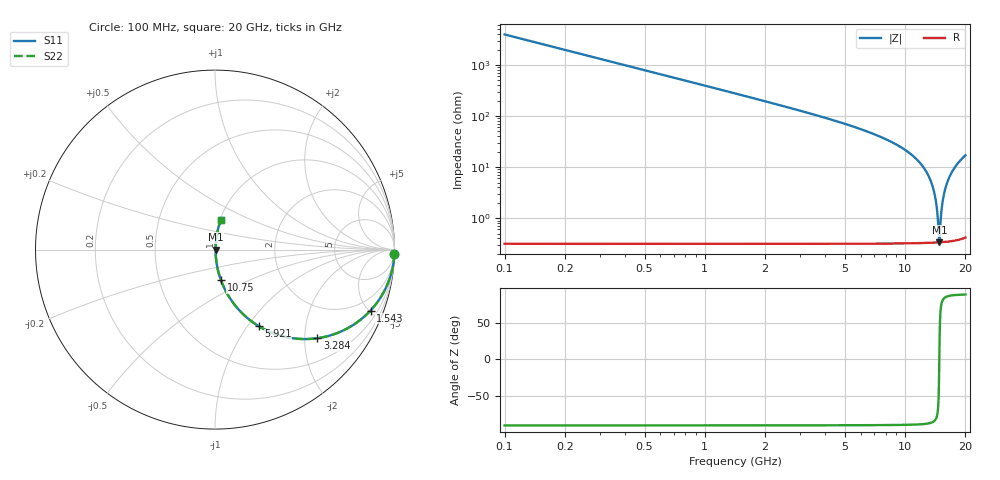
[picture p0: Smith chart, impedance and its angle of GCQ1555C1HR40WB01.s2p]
!Murata Part Number: GCQ1555C1HR40WB01
!These Parameters are Measured in Series Mode Connection
!Data Generated on Jan 08, 2026
!  o--ll--o
!Port1  Port2
!  o------o
!Operation Temp=25[degC], DC Bias Voltage=0[V]
!Freq. Start=100[MHz] Stop=20[GHz] 401[Steps]
# Hz S RI R 50
!Freq.(Hz) S11(Real) S11(Imag) S21(Real) S21(Imag) S12(Real) S12(Imag) S22(Real) S22(Imag)
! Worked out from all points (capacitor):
!   401 points, 100 MHz to 20 GHz, reference 50 ohm
!   read as one part in series: C = 400 fF near 199.5 MHz
!   lowest |Z| = 338 mohm at 14.83 GHz (marker M1)
!   series resonance near 14.82 GHz, so ESL is about 290 pH
!   S11 on the Smith chart (normalised r, x): 100 MHz: 1, -80; 1.543 GHz: 1.01, -5.10; 3.284 GHz: 1.01, -2.31; 5.921 GHz: 1.01, -1.13; 10.75 GHz: 1.01, -0.35; 20 GHz: 1.01, +0.34
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1e8  0.9994 -0.0251  0.000633 0.0251  0.000633 0.0251  0.9994 -0.0251
3.4875e8  0.9923 -0.087  0.00766 0.087  0.00766 0.087  0.9923 -0.087
5.975e8  0.9778 -0.1471  0.0222 0.1471  0.0222 0.1471  0.9778 -0.1471
1.54275e9  0.8665 -0.3395  0.1335 0.3395  0.1335 0.3395  0.8665 -0.3395
3.284e9  0.5704 -0.4937  0.4296 0.4937  0.4296 0.4937  0.5704 -0.4937
3.43325e9  0.5462 -0.4964  0.4538 0.4964  0.4538 0.4964  0.5462 -0.4964
5.92075e9  0.2437 -0.4265  0.7563 0.4265  0.7563 0.4265  0.2437 -0.4265
6.7665e9  0.1804 -0.3811  0.8196 0.3811  0.8196 0.3811  0.1804 -0.3811
1.005e10  0.0469 -0.2042  0.9531 0.2042  0.9531 0.2042  0.0469 -0.2042
1.07465e10  0.0332 -0.1702  0.9668 0.1702  0.9668 0.1702  0.0332 -0.1702
1.228875e10  0.0134 -0.1003  0.9866 0.1003  0.9866 0.1003  0.0134 -0.1003
1.338325e10  0.00631 -0.0548  0.9937 0.0548  0.9937 0.0548  0.00631 -0.0548
1.427875e10  0.00373 -0.02  0.9963 0.02  0.9963 0.02  0.00373 -0.02
1.45275e10  0.00345 -0.0106  0.9965 0.0106  0.9965 0.0106  0.00345 -0.0106
1.47265e10  0.00336 -0.00329  0.9966 0.00329  0.9966 0.00329  0.00336 -0.00329
1.4826e10  0.00335 0.000358  0.9966 -0.000358  0.9966 -0.000358  0.00335 0.000358
1.517425e10  0.00354 0.0129  0.9965 -0.0129  0.9965 -0.0129  0.00354 0.0129
1.547275e10  0.00395 0.0235  0.9961 -0.0235  0.9961 -0.0235  0.00395 0.0235
1.597025e10  0.0051 0.0407  0.9949 -0.0407  0.9949 -0.0407  0.0051 0.0407
1.67165e10  0.00784 0.0656  0.9922 -0.0656  0.9922 -0.0656  0.00784 0.0656
1.81095e10  0.0159 0.1095  0.9841 -0.1095  0.9841 -0.1095  0.0159 0.1095
2e10  0.0321 0.1646  0.9679 -0.1646  0.9679 -0.1646  0.0321 0.1646
